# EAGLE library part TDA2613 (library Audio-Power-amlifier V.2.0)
6 W hi-fi audio power amplifier Philips Semiconductors
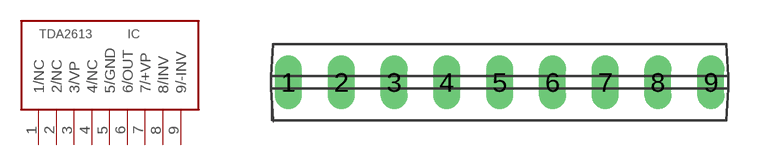
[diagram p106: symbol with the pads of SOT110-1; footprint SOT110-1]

Designator prefix IC

## TDA2613  [SOT110-1]
1  1/NC  nc
2  2/NC  nc
3  3/VP  in
4  4/NC  nc
5  5/GND  pwr
6  6/OUT  out
7  7/+VP  pwr
8  8/INV  in
9  9/-INV  in

## Footprint SOT110-1 (pad centres in mm)
SIL9MPF: plastic single in-line medium power package with fin; 9 leads
drill 0.8 long: 1 -10.16,0; 2 -7.62,0; 3 -5.08,0; 4 -2.54,0; 5 0,0; 6 2.54,0; 7 5.08,0; 8 7.62,0; 9 10.16,0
